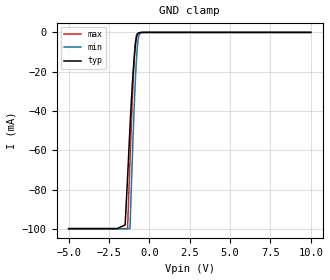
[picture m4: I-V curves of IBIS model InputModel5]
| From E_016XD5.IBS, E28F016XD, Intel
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|*******************Input Model 5*************************************
[Model]   InputModel5
Model_type   Input
|   for pin29(NC), pin30(NC)
Vinl = 0.8V
Vinh = 2.0V
|Variable   typ   min   max
C_comp   5.61p   NA   7.6p
[Voltage Range]   5.0V   4.5V   5.5V
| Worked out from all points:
|   GND clamp passes 1 mA (typ) near -0.74 V on its own axis
[GND_clamp]
|Voltage I(typ)   I(min)   I(max)
-5V       -99.85mA   -99.85mA   -99.85mA
-2V       -99.85mA   -99.85mA   -99.85mA
-1.5V     -97.95mA   -99.85mA   -99.85mA
-1.35V    -73.97mA   -99.85mA   -99.85mA
-1.2V     -48.56mA   -99.73mA   -65.75mA
-1.05V    -26.05mA   -63.01mA   -33.82mA
-950mV    -14.23mA   -40.6mA    -15.79mA
-850mV    -5.527mA   -21.59mA   -4.036mA
-750mV    -1.162mA   -7.935mA   -647.2uA
-650mV    -288.6uA   -1.837mA   -234.7uA
-500mV    -44.36uA   0A         -28.02uA
10V       0A         0A         0A
[POWER_clamp]
| Input buffer circuits of this product do not intrinsically
| require a [POWER_clamp] definition.  This zero current
| [POWER_clamp] is provided for compatibility with some ibis
| parsers.
|Voltage  I(typ)   I(min)   I(max)
-5V       0A         0A         0A
0V        0A         0A         0A
5V        0A         0A         0A
10V       0A         0A         0A
